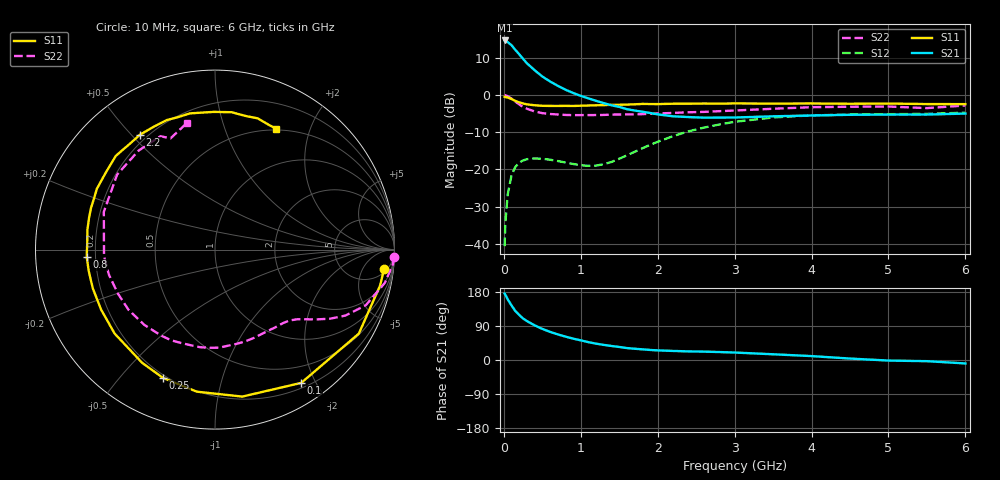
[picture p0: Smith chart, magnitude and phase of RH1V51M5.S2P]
! SIEMENS Small Signal Semiconductors
! BFR106
! Si NPN RF Bipolar Junction Transistor in SOT23
! VCE = 1.5 V  IC = 1.5 mA
! Common Emitter S-Parameters:  August  1996
# GHz  S  MA  R  50
!  f  S11  S21  S12  S22
! GHz  MAG  ANG  MAG  ANG  MAG  ANG  MAG  ANG
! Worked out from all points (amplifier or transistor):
!   36 points, 10 MHz to 6 GHz, reference 50 ohm
!   highest |S21| = 14.7 dB at 10 MHz (marker M1)
!   |S21| within 3 dB of that: start of sweep to 169.3 MHz
!   unconditionally stable (mu >= 1): 805 MHz to end of sweep
!   at 250 MHz: K = 0.30, MSG = 13.7 dB, |S12| = -17.6 dB
!   at 1.4 GHz: K = 1.39, MAG = 3.9 dB, |S12| = -18.0 dB
!   at 6 GHz: K = 1.02, MAG = -1.0 dB, |S12| = -4.7 dB
!   S11 on the Smith chart (normalised r, x): 10 MHz: 7, -15; 100 MHz: 0.27, -1.81; 250 MHz: 0.19, -0.66; 800 MHz: 0.17, -0.03; 2.2 GHz: 0.17, +0.53; 6 GHz: 0.48, +1.51
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0.01  0.9487 -6.4  5.421 175.3  0.0093 87.2  0.9979 -2.4
0.02  0.9411 -12.4  5.364 172.2  0.0192 83.0  0.995 -4.6
0.05  0.928 -30.3  5.161 160.1  0.0462 72.9  0.9643 -11.1
0.1  0.8844 -57.1  4.672 144.0  0.0838 58.8  0.8952 -20.3
0.15  0.8329 -79.5  4.039 129.1  0.1082 46.9  0.8146 -26.8
0.2  0.798 -97.3  3.537 118.8  0.1233 39.0  0.7492 -30.9
0.25  0.7715 -112.0  3.068 109.4  0.1322 32.1  0.6914 -34.2
0.3  0.75 -122.8  2.678 102.7  0.1373 28.1  0.6547 -36.4
0.4  0.7291 -140.1  2.158 91.5  0.1407 21.4  0.6021 -40.1
0.5  0.7172 -152.2  1.779 82.1  0.1391 17.7  0.5713 -43.8
0.6  0.7142 -162.3  1.524 74.3  0.1351 15.9  0.5565 -47.7
0.8  0.7159 -176.7  1.181 61.8  0.1239 16.9  0.5407 -56.6
1.1  0.7236 165.9  0.902 47.1  0.1119 29.5  0.5382 -71.6
1.6  0.7449 144.5  0.646 31.5  0.1546 57.2  0.5502 -98.7
2.2  0.7645 123.1  0.518 23.9  0.2805 58.6  0.5752 -133.1
2.8  0.7664 105.3  0.498 21.0  0.4021 46.1  0.6072 -166.7
3.5  0.7673 90.6  0.518 15.1  0.4997 29.6  0.6543 161.2
4  0.771 83.1  0.531 10.3  0.5334 19.0  0.6871 142.5
4.5  0.7637 76.8  0.543 3.8  0.5466 10.1  0.6966 127.7
5  0.769 72.0  0.547 -1.5  0.5533 3.0  0.7012 115.7
5.5  0.7567 66.5  0.547 -3.1  0.5588 -0.3  0.6674 111.8
6  0.7552 63.3  0.564 -9.1  0.5796 -7.6  0.7242 102.3
